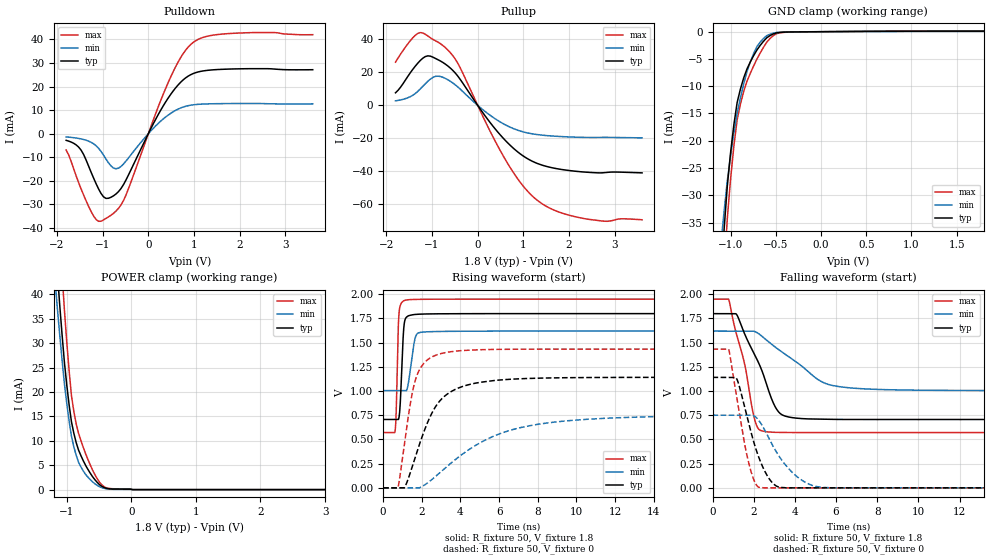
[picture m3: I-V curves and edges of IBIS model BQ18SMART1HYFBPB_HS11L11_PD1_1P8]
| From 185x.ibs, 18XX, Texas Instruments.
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|   Model Cell BQ18SMART1HYFBPB_HS11L11_PD1_1P8
|BQ18SMART1HYFBPB_HS11L11_PD1_1P8
[Model]   BQ18SMART1HYFBPB_HS11L11_PD1_1P8
Model_type   I/O
Polarity   Non-Inverting
Enable   Active-Low
Vinl =  0.63
Vinh =  1.17
Cref =  15pF
Rref =  100.0000M
Vref =  0V
Vmeas =  0.9
C_comp   0.915143p   0.8088923p   1.028577p
[Model Spec]
Vinl   0.63   0.567   0.6825
Vinh   1.17   1.053   1.2675
[Temperature Range]   25   125   -40
[Voltage Range]   1.8   1.62   1.95
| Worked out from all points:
|   slope of the pulldown table from 0 to 0.27 V, typ, clamps not added: 27.2 ohm
|   slope of the pullup table from 0 to 0.27 V, typ, clamps not added: 26 ohm
|   GND clamp passes 1 mA (typ) near -0.59 V on its own axis
|   POWER clamp passes 1 mA (typ) near -0.49 V on its own axis
|   rising waveform, R_fixture 50, V_fixture 1.8: 20-80 % time 144ps typ, 262ps min, 101ps max; typ from 0.706 V to 1.8 V
|   rising waveform, R_fixture 50, V_fixture 0: 20-80 % time 1.48ns typ, 3.7ns min, 736ps max; typ from 0 V to 1.14 V
|   falling waveform, R_fixture 50, V_fixture 1.8: 20-80 % time 1.28ns typ, 2.27ns min, 843ps max; typ from 1.8 V to 0.706 V
|   falling waveform, R_fixture 50, V_fixture 0: 20-80 % time 944ps typ, 1.39ns min, 712ps max; typ from 1.14 V to 0 V
| Nom Voltages:
|   BIASFET=1.8, VBBNW=1.1, VDD=1.1, VDDS=1.8, VSS=0, VSSS=0
| Min Voltages:
|   BIASFET=1.62, VBBNW=0.99, VDD=0.99, VDDS=1.62, VSS=0, VSSS=0
| Max Voltages:
|   BIASFET=1.95, VBBNW=1.21, VDD=1.21, VDDS=1.95, VSS=0, VSSS=0
[POWER_clamp]
|   voltage   I(typ)   I(min)   I(max)
-1.8V     196.9mA    157.5mA    250.4mA
-1.182V   51.67mA    43mA       68.61mA
-1.145V   44.45mA    37.16mA    60.1mA
-1.109V   37.9mA     31.74mA    52.07mA
-1.073V   31.79mA    26.6mA     44.33mA
-1.036V   26.12mA    21.74mA    36.87mA
-963.6mV  17.39mA    14.07mA    24.42mA
-927.3mV  13.91mA    10.96mA    19.29mA
-854.5mV  9.657mA    7.054mA    13.5mA
-709.1mV  4.995mA    3.131mA    7.393mA
-490.9mV  991uA      585.4uA    1.466mA
3.6V      0A         0A         0A
[Pulldown]
|   voltage   I(typ)   I(min)   I(max)
-1.8V     -2.835mA   -1.376mA   -6.938mA
-1.473V   -6.994mA   -2.229mA   -23.44mA
-1.2V     -18.79mA   -4.282mA   -34.89mA
-1.036V   -25.34mA   -7.531mA   -37.14mA
-872.7mV  -27.39mA   -12.36mA   -35.28mA
-654.5mV  -24.59mA   -14.63mA   -31.68mA
-490.9mV  -19.69mA   -11.65mA   -26.08mA
381.8mV   13.54mA    7.116mA    19.32mA
654.5mV   20.72mA    10.44mA    30.47mA
927.3mV   25mA       12.07mA    37.79mA
1.636V    27.3mA     12.74mA    42.26mA
3.6V      27.12mA    12.64mA    41.97mA
[Pullup]
|   voltage   I(typ)   I(min)   I(max)
-1.8V     7.614mA    2.74mA     26.22mA
-1.527V   17.69mA    4.626mA    37.43mA
-1.309V   25.69mA    8.541mA    43.72mA
-1.036V   29.87mA    15.94mA    41.05mA
-818.2mV  26.95mA    17.52mA    37.49mA
-490.9mV  19.61mA    12.45mA    28.08mA
545.5mV   -19.54mA   -10.94mA   -30.03mA
927.3mV   -29.38mA   -15.56mA   -46.58mA
1.255V    -34.7mA    -17.56mA   -56.51mA
1.691V    -38.25mA   -18.74mA   -63.85mA
2.291V    -40.42mA   -19.45mA   -68.55mA
3.6V      -41.01mA   -19.75mA   -69.5mA
[GND_clamp]
|   voltage   I(typ)   I(min)   I(max)
-1.8V     -274mA     -200.4mA   -365.5mA
-1.109V   -45.41mA   -39.33mA   -55.91mA
-1.073V   -36.49mA   -33.11mA   -44.46mA
-1.036V   -28.34mA   -27.37mA   -34.29mA
-1V       -22.19mA   -22.71mA   -27mA
-927.3mV  -12.97mA   -14.93mA   -16.12mA
-854.5mV  -8.452mA   -9.555mA   -10.93mA
-781.8mV  -5.549mA   -5.539mA   -7.634mA
-709.1mV  -3.363mA   -2.741mA   -5.028mA
-600mV    -1.121mA   -737.1uA   -1.924mA
-381.8mV  -62.21uA   -38.42uA   -93.33uA
1.8V      98.66uA    51.35uA    168.2uA
[Ramp]
| variable   typ   min   max
dV/dt_f 0.65747079/1.2836838n 0.37042735/2.2804984n 0.82860283/0.84564035n
dV/dt_r 0.69356081/1.4868665n   0.457084/3.7995356n 0.86806978/0.73882422n
R_load = 50
[Rising Waveform]
R_fixture = 50
V_fixture = 1.8
V_fixture_min = 1.62
V_fixture_max = 1.95
|   time   V(typ)   V(min)   V(max)
0s        706.1mV    1.004V     571mV
614.5ps   706.1mV    1.004V     584.7mV
669.8ps   706.1mV    1.004V     753.9mV
765.9ps   706.1mV    1.004V     1.554V
813.1ps   720.6mV    1.004V     1.784V
1.103ns   1.71V      1.004V     1.934V
1.277ns   1.772V     1.051V     1.941V
1.667ns   1.79V      1.553V     1.945V
1.934ns   1.793V     1.605V     1.946V
17.87ns   1.798V     1.619V     1.948V
[Rising Waveform]
R_fixture = 50
V_fixture = 0
V_fixture_min = 0
V_fixture_max = 0
|   time   V(typ)   V(min)   V(max)
0s        0V         0V         0V
765.1ps   0V         0V         0V
1.098ns   0V         0V         454.8mV
1.405ns   156.7mV    0V         867mV
1.644ns   305.9mV    0V         1.097V
2.019ns   530.6mV    14.9mV     1.263V
2.684ns   829.1mV    112.9mV    1.366V
4.164ns   1.05V      356.9mV    1.418V
7.352ns   1.128V     632.2mV    1.431V
18.03ns   1.141V     743.9mV    1.432V
[Falling Waveform]
R_fixture = 50
V_fixture = 1.8
V_fixture_min = 1.62
V_fixture_max = 1.95
|   time   V(typ)   V(min)   V(max)
0s        1.798V     1.618V     1.948V
797ps     1.798V     1.618V     1.939V
1.189ns   1.784V     1.618V     1.568V
1.583ns   1.578V     1.618V     1.255V
2.022ns   1.385V     1.616V     725.7mV
2.339ns   1.242V     1.576V     592.7mV
3.09ns    819.9mV    1.446V     573mV
3.811ns   727.1mV    1.338V     571.2mV
6.445ns   706.1mV    1.037V     571mV
17.87ns   705.8mV    1.004V     571mV
[Falling Waveform]
R_fixture = 50
V_fixture = 0
V_fixture_min = 0
V_fixture_max = 0
|   time   V(typ)   V(min)   V(max)
0s        1.141V     750.3mV    1.432V
797ps     1.141V     750.3mV    1.422V
1.189ns   1.12V      750.3mV    920.5mV
1.657ns   752.8mV    750.3mV    351.7mV
1.986ns   485.6mV    746.8mV    94.23mV
2.251ns   313.6mV    695.6mV    6.308mV
3.127ns   15.82mV    361.9mV    0V
4.093ns   0V         117.6mV    0V
5.019ns   0V         15.01mV    0V
18.03ns   0V         0V         0V
